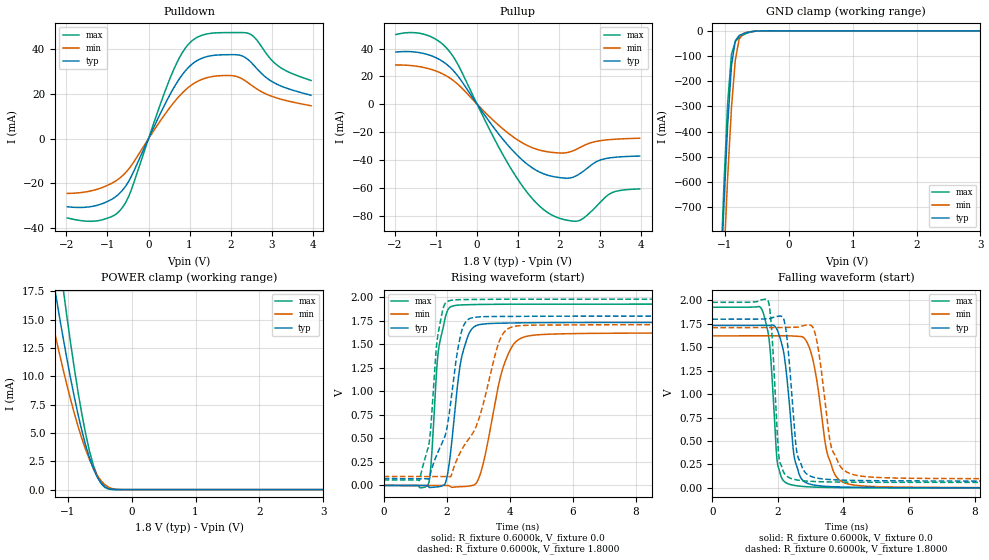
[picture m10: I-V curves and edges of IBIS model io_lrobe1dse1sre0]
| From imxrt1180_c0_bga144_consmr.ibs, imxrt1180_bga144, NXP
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[Model]  io_lrobe1dse1sre0
|   Model io_lrobe1dse1sre0
| This model was characterised for following simulation conditions:
| External (pad) voltage:
|   - Typ: 1.8V,   - Min: 1.71V,   - Max: 1.98V
| Library cells for typ/min/max conditions are connected as defined below:
|  PAD_IO - External Pad
|  ipp_do - Core Input
|  ipp_obe - Output Buffer Enable
|  ASRCN3V3[3] - NC
|  ASRCN3V3[4] - NC
|  ASRCP3V3[4] - NC
|  REFAPBIAS3V3 - gnde
|  REFBAMPL3V3 - vdd1v8
|  REFCAMPH3V3 - vdd1v8
|  REFDNBIAS3V3 - vdd1v8
|  REFH3V3 - REFH3V3
|  REFL3V3 - REFL3V3
|  gnde - gnde
|  ipp_dse - vdd
|  ipp_ina235_3v - NC
|  ipp_ina40_3v - NC
|  ipp_ina_mux - NC
|  ipp_ind - NC
|  ipp_ind_1p8v - NC
|  ipp_ind_3v - NC
|  ipp_sre - gnde
|  vdd - vdd
|  vdd1v8 - vdd1v8
|  vdda - vdde3v3
|  vdde3v3 - vdde3v3
| All other pins connected to ground
Model_type I/O
Polarity   Non-Inverting
Enable   Active-High
Vinl =   0.5400V
Vinh =   1.2600V
Vmeas =  0.9000V
Cref =   15.0000pF
Rref =   0.6000k
Vref =   0.0V
C_comp   3.9800pF   3.7960pF   4.1051pF
|C_comp_pullup   0.3211pF   0.4285pF   0.2794pF
|C_comp_pulldown   2.2498pF   2.3232pF   2.0509pF
[Model Spec]
| variable   typ   min   max
Vinh   1.2600V   NA   NA
Vinl   0.5400V   NA   NA
Vref   0.0V   0.0V   0.0V
Cref   15.0000pF   15.0000pF   15.0000pF
Rref   0.6000k   0.6000k   0.6000k
[Receiver Thresholds]
Vcross_high  =   0.0V
Vcross_low  =   0.0V
Vdiff_ac  =   0.0V
Vdiff_dc  =   0.0V
Tdiffslew_ac  =   0.0S
[Temperature Range]   25.0000   0.1250k   -40.0000
[Voltage Range]   1.8000V   1.7100V   1.9800V
[Pullup Reference]   1.8000V   1.7100V   1.9800V
[Pulldown Reference]   0.0V   0.0V   0.0V
[POWER Clamp Reference]   1.8000V   1.7100V   1.9800V
[GND Clamp Reference]   0.0V   0.0V   0.0V
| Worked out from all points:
|   slope of the pulldown table from 0 to 0.27 V, typ, clamps not added: 25.6 ohm
|   slope of the pullup table from 0 to 0.27 V, typ, clamps not added: 23.7 ohm
|   GND clamp passes 1 mA (typ) near -0.50 V on its own axis
|   POWER clamp passes 1 mA (typ) near -0.53 V on its own axis
|   rising waveform, R_fixture 0.6000k, V_fixture 0.0: 20-80 % time 368ps typ, 614ps min, 256ps max; typ from 0 V to 1.73 V
|   rising waveform, R_fixture 0.6000k, V_fixture 1.8000: 20-80 % time 548ps typ, 993ps min, 279ps max; typ from 0.072 V to 1.8 V
|   falling waveform, R_fixture 0.6000k, V_fixture 0.0: 20-80 % time 288ps typ, 435ps min, 208ps max; typ from 1.73 V to 0 V
|   falling waveform, R_fixture 0.6000k, V_fixture 1.8000: 20-80 % time 244ps typ, 371ps min, 177ps max; typ from 1.8 V to 0.072 V
[Pulldown]
|Voltage   I(typ)   I(min)   I(max)
-1.98V    -30.4mA    -24.44mA   -35.4mA
-1.2V     -29.49mA   -22.29mA   -36.54mA
-840mV    -26.45mA   -19.34mA   -34.25mA
-600mV    -22.26mA   -15.94mA   -29.79mA
-420mV    -16.87mA   -12.03mA   -22.87mA
600mV     22.22mA    15.79mA    30.28mA
900mV     30.36mA    21.79mA    40.52mA
1.14V     34.39mA    25.07mA    44.8mA
1.98V     37.52mA    28.21mA    47.38mA
2.46V     34.79mA    24.52mA    46.86mA
3.12V     24.41mA    18.2mA     33.05mA
3.96V     19.38mA    14.72mA    25.98mA
[Pullup]
|Voltage   I(typ)   I(min)   I(max)
-1.98V    37.48mA    28.19mA    50.1mA
-1.26V    36.17mA    26.14mA    50mA
-720mV    28.12mA    19.85mA    39.61mA
-480mV    20.68mA    14.63mA    29.2mA
840mV     -32.44mA   -22.67mA   -46.99mA
1.32V     -45.27mA   -30.96mA   -67.03mA
1.74V     -51.2mA    -34.29mA   -78.26mA
2.22V     -53.17mA   -34.57mA   -83.53mA
2.46V     -50.7mA    -31.84mA   -83.91mA
2.88V     -41.76mA   -26.86mA   -74.2mA
3.24V     -38.54mA   -25.42mA   -64.28mA
3.96V     -37.26mA   -24.44mA   -60.88mA
[GND_clamp]
|Voltage   I(typ)   I(min)   I(max)
-1.98V    -7.543A    -7.6A      -7.897A
-1.08V    -1.077A    -1.286A    -1.025A
-1.02V    -705.3mA   -921.3mA   -628.8mA
-960mV    -377.1mA   -587.4mA   -291.7mA
-900mV    -139.2mA   -307mA     -94.38mA
-840mV    -40.12mA   -117mA     -42.82mA
-780mV    -18.81mA   -33.95mA   -26.13mA
-720mV    -11.86mA   -11.44mA   -16.78mA
-660mV    -7.061mA   -5.737mA   -9.992mA
-540mV    -1.684mA   -1.901mA   -2.15mA
-420mV    -207.1uA   -403.7uA   -160.6uA
3.96V     0A         0A         0A
[POWER_clamp]
|Voltage   I(typ)   I(min)   I(max)
-1.98V    46.79mA    35.95mA    61.44mA
-1.32V    21.78mA    16.85mA    28.96mA
-1.2V     17.57mA    13.71mA    23.37mA
-1.08V    13.59mA    10.75mA    18.03mA
-1.02V    11.71mA    9.354mA    15.49mA
-900mV    8.21mA     6.76mA     10.75mA
-720mV    3.899mA    3.511mA    4.896mA
-600mV    1.839mA    1.889mA    2.143mA
-540mV    1.103mA    1.267mA    1.197mA
-420mV    244.5uA    429.3uA    190.7uA
-180mV    281nA      5.273uA    27.6nA
3.96V     0A         0A         0A
[Ramp]
| variable   typ   min   max
dV/dt_r  1.0397/0.3678n   0.9731/0.6136n   1.1565/0.2557n
dV/dt_f  1.0366/0.2436n   0.9689/0.3707n   1.1528/0.1768n
R_load = 0.6000k
[Rising Waveform]
R_fixture= 0.6000k
V_fixture= 0.0
V_fixture_min= 0.0
V_fixture_max= 0.0
|time   V(typ)   V(min)   V(max)
0s        48.77nV    1.315uV    52.41nV
1.423ns   -12.23mV   -406.6uV   16.4mV
1.745ns   -13.7mV    -505.6uV   1.456V
2.017ns   99.71mV    36.55uV    1.852V
2.344ns   1.066V     -15.28mV   1.916V
2.86ns    1.683V     4.076mV    1.922V
3.13ns    1.714V     193.6mV    1.924V
3.962ns   1.726V     1.404V     1.926V
4.905ns   1.73V      1.601V     1.927V
60ns      1.733V     1.622V     1.927V
[Rising Waveform]
R_fixture= 0.6000k
V_fixture= 1.8000
V_fixture_min= 1.7100
V_fixture_max= 1.9800
|time   V(typ)   V(min)   V(max)
0s        72.28mV    95.11mV    58.66mV
1.139ns   71.88mV    95.03mV    55.97mV
1.453ns   85.92mV    94.65mV    473.6mV
1.663ns   307.1mV    94.6mV     1.436V
1.834ns   437mV      94.8mV     1.808V
2.227ns   1.149V     191.7mV    1.971V
2.651ns   1.756V     471.6mV    1.976V
3.692ns   1.796V     1.553V     1.979V
4.318ns   1.797V     1.698V     1.979V
60ns      1.8V       1.71V      1.98V
[Falling Waveform]
R_fixture= 0.6000k
V_fixture= 0.0
V_fixture_min= 0.0
V_fixture_max= 0.0
|time   V(typ)   V(min)   V(max)
0s        1.733V     1.622V     1.927V
1.525ns   1.734V     1.622V     1.894V
1.752ns   1.733V     1.621V     1.518V
1.948ns   1.706V     1.622V     410.2mV
2.179ns   1.441V     1.623V     72.99mV
2.691ns   112.2mV    1.617V     17.09mV
3.049ns   33.06mV    1.393V     8.975mV
3.683ns   11.95mV    184.4mV    3.517mV
4.534ns   5.197mV    21.61mV    1.215mV
60ns      2.967uV    6.179uV    1.433uV
[Falling Waveform]
R_fixture= 0.6000k
V_fixture= 1.8000
V_fixture_min= 1.7100
V_fixture_max= 1.9800
|time   V(typ)   V(min)   V(max)
0s        1.8V       1.71V      1.98V
1.71ns    1.804V     1.71V      1.989V
2.021ns   1.833V     1.71V      367.7mV
2.156ns   1.818V     1.711V     182.7mV
2.555ns   436.8mV    1.715V     86mV
2.784ns   187mV      1.732V     75.14mV
3.166ns   106mV      1.605V     66.92mV
3.66ns    86.8mV     399.6mV    62.58mV
4.771ns   76.88mV    116.8mV    59.63mV
60ns      72.29mV    95.11mV    58.66mV
